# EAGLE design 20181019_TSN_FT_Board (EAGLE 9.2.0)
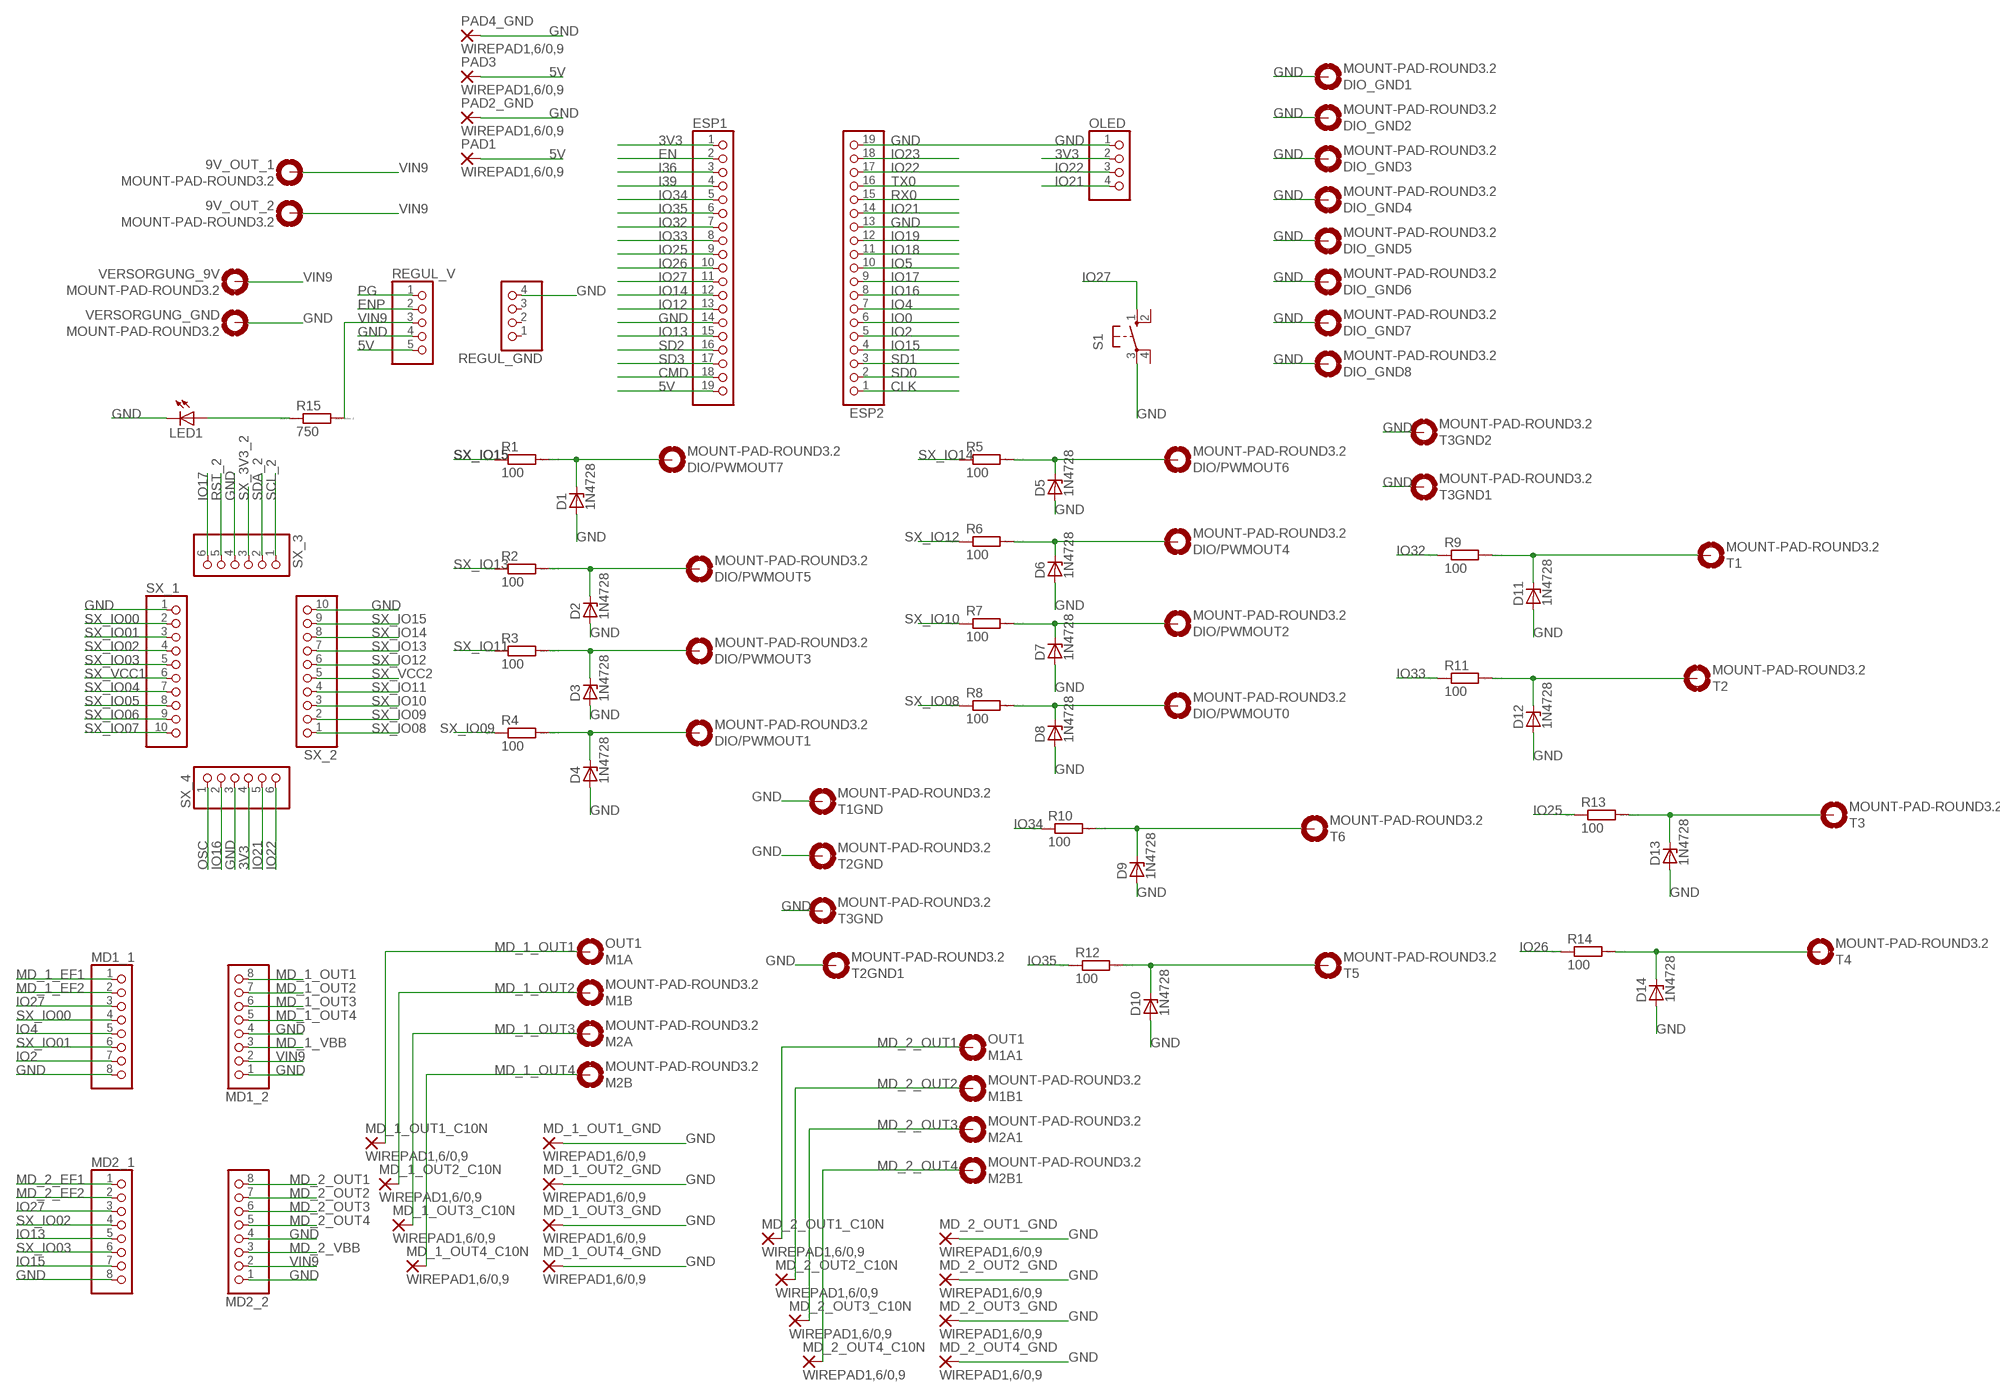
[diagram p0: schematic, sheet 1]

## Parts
9V_OUT_1  MOUNT-PAD-ROUND3.2  [3,2-PAD]
9V_OUT_2  MOUNT-PAD-ROUND3.2  [3,2-PAD]
D1  1N4728  [DO41Z10]
D2  1N4728  [DO41Z10]
D3  1N4728  [DO41Z10]
D4  1N4728  [DO41Z10]
D5  1N4728  [DO41Z10]
D6  1N4728  [DO41Z10]
D7  1N4728  [DO41Z10]
D8  1N4728  [DO41Z10]
D9  1N4728  [DO41Z10]
D10  1N4728  [DO41Z10]
D11  1N4728  [DO41Z10]
D12  1N4728  [DO41Z10]
D13  1N4728  [DO41Z10]
D14  1N4728  [DO41Z10]
DIO/PWMOUT0  MOUNT-PAD-ROUND3.2  [3,2-PAD]
DIO/PWMOUT1  MOUNT-PAD-ROUND3.2  [3,2-PAD]
DIO/PWMOUT2  MOUNT-PAD-ROUND3.2  [3,2-PAD]
DIO/PWMOUT3  MOUNT-PAD-ROUND3.2  [3,2-PAD]
DIO/PWMOUT4  MOUNT-PAD-ROUND3.2  [3,2-PAD]
DIO/PWMOUT5  MOUNT-PAD-ROUND3.2  [3,2-PAD]
DIO/PWMOUT6  MOUNT-PAD-ROUND3.2  [3,2-PAD]
DIO/PWMOUT7  MOUNT-PAD-ROUND3.2  [3,2-PAD]
DIO_GND1  MOUNT-PAD-ROUND3.2  [3,2-PAD]
DIO_GND2  MOUNT-PAD-ROUND3.2  [3,2-PAD]
DIO_GND3  MOUNT-PAD-ROUND3.2  [3,2-PAD]
DIO_GND4  MOUNT-PAD-ROUND3.2  [3,2-PAD]
DIO_GND5  MOUNT-PAD-ROUND3.2  [3,2-PAD]
DIO_GND6  MOUNT-PAD-ROUND3.2  [3,2-PAD]
DIO_GND7  MOUNT-PAD-ROUND3.2  [3,2-PAD]
DIO_GND8  MOUNT-PAD-ROUND3.2  [3,2-PAD]
ESP1  PINHD-1X19  [1X19]
ESP2  PINHD-1X19  [1X19]
LED1  LED3MM  [LED3MM]
M1A  OUT1  MOUNT-PAD-ROUND3.2  [3,2-PAD]
M1A1  OUT1  MOUNT-PAD-ROUND3.2  [3,2-PAD]
M1B  MOUNT-PAD-ROUND3.2  [3,2-PAD]
M1B1  MOUNT-PAD-ROUND3.2  [3,2-PAD]
M2A  MOUNT-PAD-ROUND3.2  [3,2-PAD]
M2A1  MOUNT-PAD-ROUND3.2  [3,2-PAD]
M2B  MOUNT-PAD-ROUND3.2  [3,2-PAD]
M2B1  MOUNT-PAD-ROUND3.2  [3,2-PAD]
MD1_1  PINHD-1X8  [1X08]
MD1_2  PINHD-1X8  [1X08]
MD2_1  PINHD-1X8  [1X08]
MD2_2  PINHD-1X8  [1X08]
MD_1_OUT1_C10N  WIREPAD1,6/0,9  [1,6/0,9]
MD_1_OUT1_GND  WIREPAD1,6/0,9  [1,6/0,9]
MD_1_OUT2_C10N  WIREPAD1,6/0,9  [1,6/0,9]
MD_1_OUT2_GND  WIREPAD1,6/0,9  [1,6/0,9]
MD_1_OUT3_C10N  WIREPAD1,6/0,9  [1,6/0,9]
MD_1_OUT3_GND  WIREPAD1,6/0,9  [1,6/0,9]
MD_1_OUT4_C10N  WIREPAD1,6/0,9  [1,6/0,9]
MD_1_OUT4_GND  WIREPAD1,6/0,9  [1,6/0,9]
MD_2_OUT1_C10N  WIREPAD1,6/0,9  [1,6/0,9]
MD_2_OUT1_GND  WIREPAD1,6/0,9  [1,6/0,9]
MD_2_OUT2_C10N  WIREPAD1,6/0,9  [1,6/0,9]
MD_2_OUT2_GND  WIREPAD1,6/0,9  [1,6/0,9]
MD_2_OUT3_C10N  WIREPAD1,6/0,9  [1,6/0,9]
MD_2_OUT3_GND  WIREPAD1,6/0,9  [1,6/0,9]
MD_2_OUT4_C10N  WIREPAD1,6/0,9  [1,6/0,9]
MD_2_OUT4_GND  WIREPAD1,6/0,9  [1,6/0,9]
OLED  PINHD-1X4  [1X04]
PAD1  WIREPAD1,6/0,9  [1,6/0,9]
PAD2_GND  WIREPAD1,6/0,9  [1,6/0,9]
PAD3  WIREPAD1,6/0,9  [1,6/0,9]
PAD4_GND  WIREPAD1,6/0,9  [1,6/0,9]
R1  100  R0207/10  [0207/10]
R2  100  R0207/10  [0207/10]
R3  100  R0207/10  [0207/10]
R4  100  R0207/10  [0207/10]
R5  100  R0207/10  [0207/10]
R6  100  R0207/10  [0207/10]
R7  100  R0207/10  [0207/10]
R8  100  R0207/10  [0207/10]
R9  100  R0207/10  [0207/10]
R10  100  R0207/10  [0207/10]
R11  100  R0207/10  [0207/10]
R12  100  R0207/10  [0207/10]
R13  100  R0207/10  [0207/10]
R14  100  R0207/10  [0207/10]
R15  750  R0207/10  [0207/10]
REGUL_GND  PINHD-1X4  [1X04]
REGUL_V  PINHD-1X5  [1X05]
S1  10-XX  [B3F-10XX]
SX_1  PINHD-1X10  [1X10]
SX_2  PINHD-1X10  [1X10]
SX_3  PINHD-1X6  [1X06]
SX_4  PINHD-1X6  [1X06]
T1  MOUNT-PAD-ROUND3.2  [3,2-PAD]
T1GND  MOUNT-PAD-ROUND3.2  [3,2-PAD]
T2  MOUNT-PAD-ROUND3.2  [3,2-PAD]
T2GND  MOUNT-PAD-ROUND3.2  [3,2-PAD]
T2GND1  MOUNT-PAD-ROUND3.2  [3,2-PAD]
T3  MOUNT-PAD-ROUND3.2  [3,2-PAD]
T3GND  MOUNT-PAD-ROUND3.2  [3,2-PAD]
T3GND1  MOUNT-PAD-ROUND3.2  [3,2-PAD]
T3GND2  MOUNT-PAD-ROUND3.2  [3,2-PAD]
T4  MOUNT-PAD-ROUND3.2  [3,2-PAD]
T5  MOUNT-PAD-ROUND3.2  [3,2-PAD]
T6  MOUNT-PAD-ROUND3.2  [3,2-PAD]
VERSORGUNG_9V  MOUNT-PAD-ROUND3.2  [3,2-PAD]
VERSORGUNG_GND  MOUNT-PAD-ROUND3.2  [3,2-PAD]

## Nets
3V3 [3V3]: ESP1.1 OLED.2 SX_4.4
5V [Bigger]: ESP1.19 PAD1.1(P) PAD3.1(P) REGUL_V.5
CLK: ESP2.1
CMD: ESP1.18
EN: ESP1.2
ENP: REGUL_V.2
GND [MOT_OUT]: D1.A D2.A D3.A D4.A D5.A D6.A D7.A D8.A D9.A D10.A D11.A D12.A D13.A D14.A DIO_GND1.BH3,2(MOUNT) DIO_GND2.BH3,2(MOUNT) DIO_GND3.BH3,2(MOUNT) DIO_GND4.BH3,2(MOUNT) DIO_GND5.BH3,2(MOUNT) DIO_GND6.BH3,2(MOUNT) DIO_GND7.BH3,2(MOUNT) DIO_GND8.BH3,2(MOUNT) ESP1.14 ESP2.13 ESP2.19 LED1.K(C) MD1_1.8 MD1_2.1 MD1_2.4 MD2_1.8 MD2_2.1 MD2_2.4 MD_1_OUT1_GND.1(P) MD_1_OUT2_GND.1(P) MD_1_OUT3_GND.1(P) MD_1_OUT4_GND.1(P) MD_2_OUT1_GND.1(P) MD_2_OUT2_GND.1(P) MD_2_OUT3_GND.1(P) MD_2_OUT4_GND.1(P) OLED.1 PAD2_GND.1(P) PAD4_GND.1(P) REGUL_GND.4 REGUL_V.4 S1.3(P) SX_1.1 SX_2.10 SX_3.4 SX_4.3 T1GND.BH3,2(MOUNT) T2GND1.BH3,2(MOUNT) T2GND.BH3,2(MOUNT) T3GND1.BH3,2(MOUNT) T3GND2.BH3,2(MOUNT) T3GND.BH3,2(MOUNT) VERSORGUNG_GND.BH3,2(MOUNT)
I36: ESP1.3
I39: ESP1.4
IO0: ESP2.6
IO2: ESP2.5 MD1_1.7
IO4: ESP2.7 MD1_1.5
IO5: ESP2.10
IO12: ESP1.13
IO13: ESP1.15 MD2_1.5
IO14: ESP1.12
IO15: ESP2.4 MD2_1.7
IO16: ESP2.8 SX_4.2
IO17: ESP2.9 SX_3.6
IO18: ESP2.11
IO19: ESP2.12
IO21: ESP2.14 OLED.4 SX_4.5
IO22: ESP2.17 OLED.3 SX_4.6
IO23: ESP2.18
IO25: ESP1.9 R13.1
IO26: ESP1.10 R14.1
IO27: ESP1.11 MD1_1.3 MD2_1.3 S1.1(S)
IO32: ESP1.7 R9.1
IO33: ESP1.8 R11.1
IO34: ESP1.5 R10.1
IO35: ESP1.6 R12.1
MD_1_EF1: MD1_1.1
MD_1_EF2: MD1_1.2
MD_1_OUT1 [Bigger]: M1A.BH3,2(MOUNT) MD1_2.8 MD_1_OUT1_C10N.1(P)
MD_1_OUT2 [Bigger]: M1B.BH3,2(MOUNT) MD1_2.7 MD_1_OUT2_C10N.1(P)
MD_1_OUT3 [Bigger]: M2A.BH3,2(MOUNT) MD1_2.6 MD_1_OUT3_C10N.1(P)
MD_1_OUT4 [Bigger]: M2B.BH3,2(MOUNT) MD1_2.5 MD_1_OUT4_C10N.1(P)
MD_1_VBB [MOT_OUT]: MD1_2.3
MD_2_EF1: MD2_1.1
MD_2_EF2: MD2_1.2
MD_2_OUT1 [Bigger]: M1A1.BH3,2(MOUNT) MD2_2.8 MD_2_OUT1_C10N.1(P)
MD_2_OUT2 [Bigger]: M1B1.BH3,2(MOUNT) MD2_2.7 MD_2_OUT2_C10N.1(P)
MD_2_OUT3 [Bigger]: M2A1.BH3,2(MOUNT) MD2_2.6 MD_2_OUT3_C10N.1(P)
MD_2_OUT4 [Bigger]: M2B1.BH3,2(MOUNT) MD2_2.5 MD_2_OUT4_C10N.1(P)
MD_2_VBB [MOT_OUT]: MD2_2.3
N$1: D5.C DIO/PWMOUT6.BH3,2(MOUNT) R5.2
N$2: D6.C DIO/PWMOUT4.BH3,2(MOUNT) R6.2
N$3: D7.C DIO/PWMOUT2.BH3,2(MOUNT) R7.2
N$4: D8.C DIO/PWMOUT0.BH3,2(MOUNT) R8.2
N$5: D1.C DIO/PWMOUT7.BH3,2(MOUNT) R1.2
N$6: D2.C DIO/PWMOUT5.BH3,2(MOUNT) R2.2
N$7: D3.C DIO/PWMOUT3.BH3,2(MOUNT) R3.2
N$8: D4.C DIO/PWMOUT1.BH3,2(MOUNT) R4.2
N$9: D9.C R10.2 T6.BH3,2(MOUNT)
N$10: LED1.A R15.1
N$12: D10.C R12.2 T5.BH3,2(MOUNT)
OSC: SX_4.1
PG: REGUL_V.1
RST_2: SX_3.5
RX0: ESP2.15
SCL_2: SX_3.1
SD0: ESP2.2
SD1: ESP2.3
SD2: ESP1.16
SD3: ESP1.17
SDA_2: SX_3.2
SX_3V3_2: SX_3.3
SX_IO00: MD1_1.4 SX_1.2
SX_IO01: MD1_1.6 SX_1.3
SX_IO02: MD2_1.4 SX_1.4
SX_IO03: MD2_1.6 SX_1.5
SX_IO04: SX_1.7
SX_IO05: SX_1.8
SX_IO06: SX_1.9
SX_IO07: SX_1.10
SX_IO08: R8.1 SX_2.1
SX_IO09: R4.1 SX_2.2
SX_IO10: R7.1 SX_2.3
SX_IO11: R3.1 SX_2.4
SX_IO12: R6.1 SX_2.6
SX_IO13: R2.1 SX_2.7
SX_IO14: R5.1 SX_2.8
SX_IO15: R1.1 SX_2.9
SX_IO17: D11.C R9.2 T1.BH3,2(MOUNT)
SX_IO18: D12.C R11.2 T2.BH3,2(MOUNT)
SX_IO19: D13.C R13.2 T3.BH3,2(MOUNT)
SX_IO20: D14.C R14.2 T4.BH3,2(MOUNT)
SX_VCC1: SX_1.6
SX_VCC2: SX_2.5
TX0: ESP2.16
VIN9 [MOT_OUT]: 9V_OUT_1.BH3,2(MOUNT) 9V_OUT_2.BH3,2(MOUNT) MD1_2.2 MD2_2.2 R15.2 REGUL_V.3 VERSORGUNG_9V.BH3,2(MOUNT)
Unconnected: REGUL_GND.1 REGUL_GND.2 REGUL_GND.3 S1.2(S1) S1.4(P1)

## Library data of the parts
9V_OUT_1 9V_OUT_2 DIO/PWMOUT0 DIO/PWMOUT1-DIO/PWMOUT7 DIO_GND1-DIO_GND8 M1A M1A1 M1B M1B1 M2A M2A1 M2B M2B1 T1 T1GND T2 T2GND T2GND1 T3 T3GND T3GND1 T3GND2 T4-T6 VERSORGUNG_9V VERSORGUNG_GND = Walter:MOUNT-PAD-ROUND: MOUNTING PAD, round
D1-D14 = diode:1N4728: Z DIODE
ESP1 = pinhead:PINHD-1X19: PIN HEADER
ESP2 = pinhead:PINHD-1X19: PIN HEADER; SPICEPREFIX: X
LED1 = led:LED: LED
MD1_1 MD1_2 MD2_1 MD2_2 = pinhead:PINHD-1X8: PIN HEADER
MD_1_OUT1_C10N MD_1_OUT1_GND MD_1_OUT2_C10N MD_1_OUT2_GND MD_1_OUT3_C10N MD_1_OUT3_GND MD_1_OUT4_C10N MD_1_OUT4_GND MD_2_OUT1_C10N MD_2_OUT1_GND MD_2_OUT2_C10N MD_2_OUT2_GND MD_2_OUT3_C10N MD_2_OUT3_GND MD_2_OUT4_C10N MD_2_OUT4_GND PAD1 PAD2_GND PAD3 PAD4_GND = wirepad:WIREPAD: Wire PAD connect wire on PCB
OLED REGUL_GND = pinhead:PINHD-1X4: PIN HEADER
R1-R15 = eagle-ltspice:R: RESISTOR, European symbol; SPICEMODEL: NONE; SPICEPREFIX: R
REGUL_V = pinhead:PINHD-1X5: PIN HEADER
S1 = switch-omron:10-XX: OMRON SWITCH; MPN: B3F-1000; OC_FARNELL: 176432; OC_NEWARK: 36M3542
SX_1 SX_2 = pinhead:PINHD-1X10: PIN HEADER
SX_3 SX_4 = pinhead:PINHD-1X6: PIN HEADER

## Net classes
1 MOT_OUT: width 0.6 mm
2 Bigger: width 0.6 mm
3 3V3: width 0.3 mm

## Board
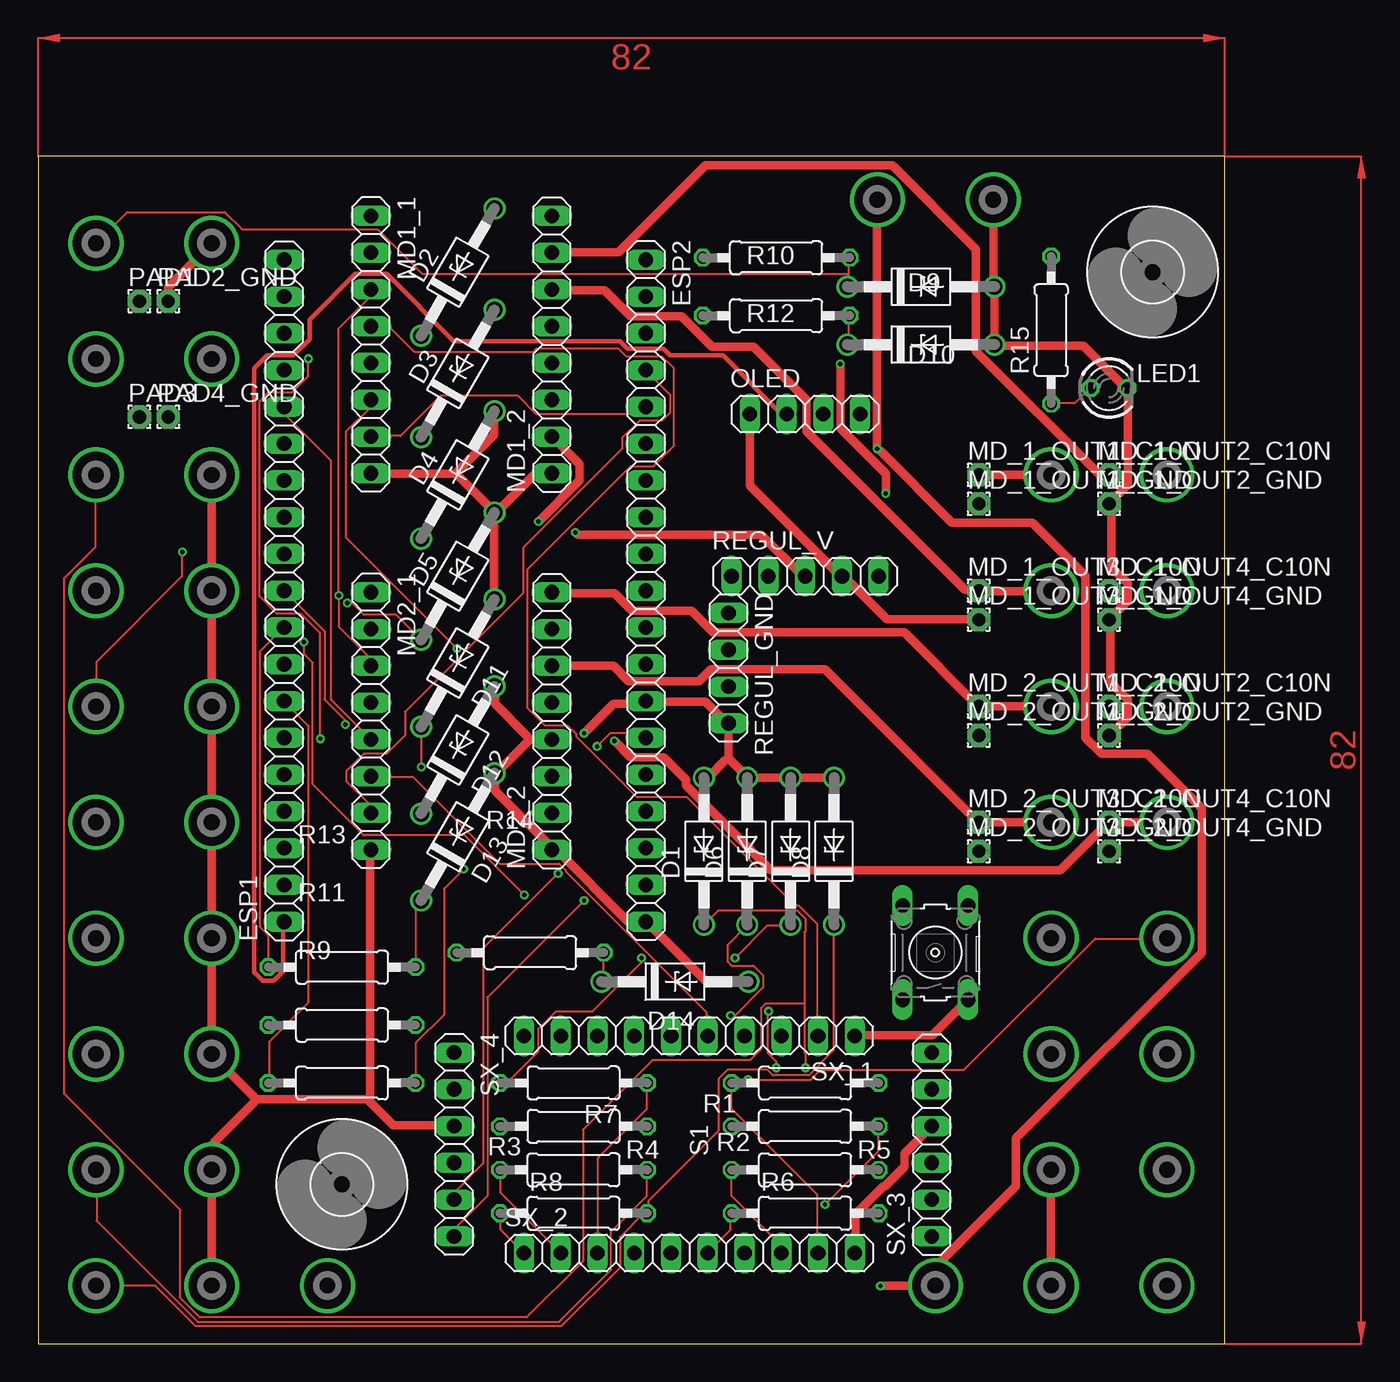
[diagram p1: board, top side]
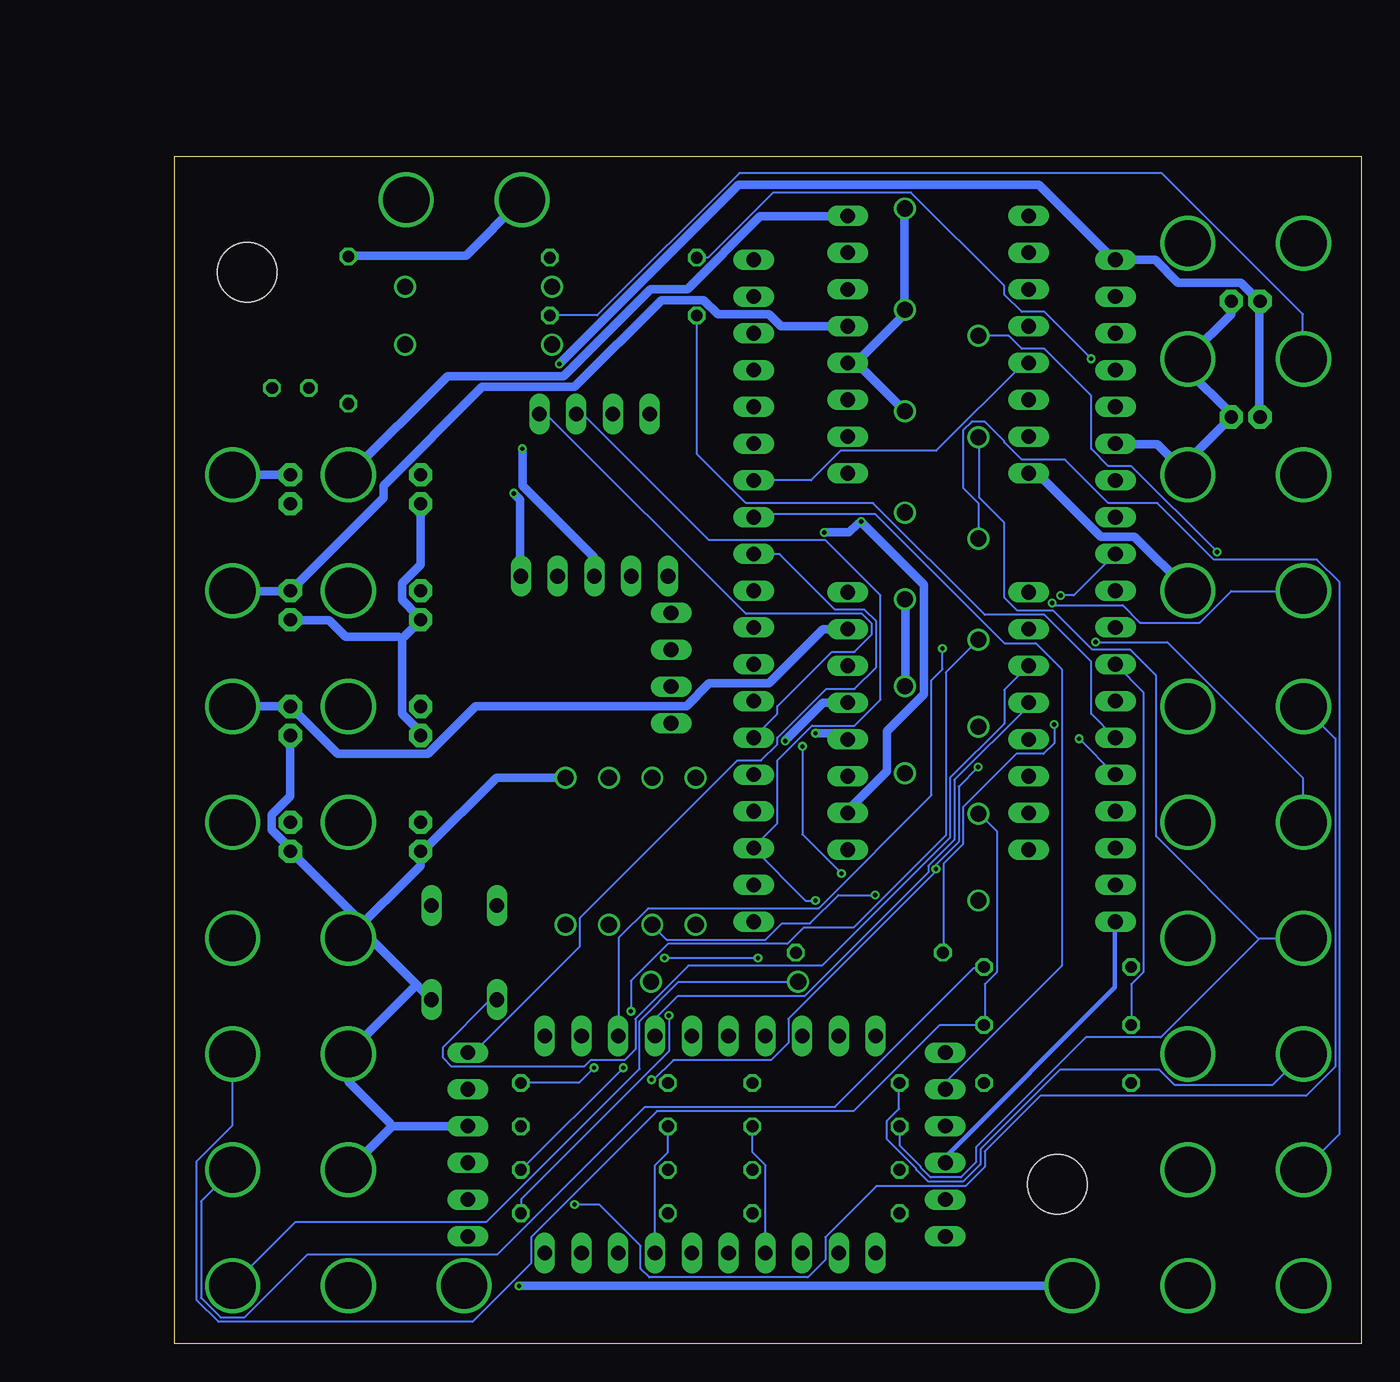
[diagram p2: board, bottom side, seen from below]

Size 82 x 82 mm. Coordinates in mm from the lower left corner, seen from the top.
Outline: 0,0 82,0 82,82 0,82 0,0
Copper layers (1+2+3*14+15+16): Top 0.035mm / dielectric 0.2mm / Route2 0.035mm / dielectric 0.36mm / Route3 0.035mm / dielectric 0.28mm / Route14 0.035mm / dielectric 0.36mm / Route15 0.035mm / dielectric 0.2mm / Bottom 0.035mm
Design rules "PCB-POOL Standard_ML6": minimum track width 0.15mm, minimum drill 0.3mm, track to track 0.15mm, track to pad 0.15mm, pad to pad 0.15mm, via to via 0.15mm, smd to smd 0.15mm, copper to edge 0.3mm, drill to drill 0.2mm, minimum pad ring 0.2mm, minimum via ring 0.15mm, stop-mask expansion 0.075mm, vias tented up to drill 0mil, thermal gap 0.2mm

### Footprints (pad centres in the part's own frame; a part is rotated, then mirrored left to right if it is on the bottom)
3,2-PAD = drill 3.2 pad 3.81: BH3,2 0,0
DO41Z10 = drill 1.118: A 5.08,0; C -5.08,0
1X19 = drill 1.016 long: 1 -22.86,0; 2 -20.32,0; 3 -17.78,0; 4 -15.24,0; 5 -12.7,0; 6 -10.16,0; 7 -7.62,0; 8 -5.08,0; 9 -2.54,0; 10 0,0; 11 2.54,0; 12 5.08,0; 13 7.62,0; 14 10.16,0; 15 12.7,0; 16 15.24,0; 17 17.78,0; 18 20.32,0; 19 22.86,0
LED3MM = drill 0.813 octagon: A -1.27,0; K 1.27,0
1X08 = drill 1.016 long: 1 -8.89,0; 2 -6.35,0; 3 -3.81,0; 4 -1.27,0; 5 1.27,0; 6 3.81,0; 7 6.35,0; 8 8.89,0
1,6/0,9 = drill 0.914 pad 1.6 octagon: 1 0,0
1X04 = drill 1.016 long: 1 -3.81,0; 2 -1.27,0; 3 1.27,0; 4 3.81,0
0207/10 = drill 0.813 octagon: 1 -5.08,0; 2 5.08,0
1X05 = drill 1.016 long: 1 -5.08,0; 2 -2.54,0; 3 0,0; 4 2.54,0; 5 5.08,0
B3F-10XX = drill 1.016 long: 1 -3.251,2.261; 2 3.251,2.261; 3 -3.251,-2.261; 4 3.251,-2.261
1X10 = drill 1.016 long: 1 -11.43,0; 2 -8.89,0; 3 -6.35,0; 4 -3.81,0; 5 -1.27,0; 6 1.27,0; 7 3.81,0; 8 6.35,0; 9 8.89,0; 10 11.43,0
1X06 = drill 1.016 long: 1 -6.35,0; 2 -3.81,0; 3 -1.27,0; 4 1.27,0; 5 3.81,0; 6 6.35,0
4,1 = hole 4.1: 0,0

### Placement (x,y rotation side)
9V_OUT_1  20,4 0 top
9V_OUT_2  62,4 0 top
D1  46,34 90 top
D2  29,74 60 top
D3  29,67 60 top
D4  29,60 60 top
D5  29,53 60 top
D6  49,34 90 top
D7  52,34 90 top
D8  55,34 90 top
D9  61,73 0 top
D10  61,69 0 top
D11  29,47 60 top
D12  29,41 60 top
D13  29,35 60 top
D14  44,25 0 top
DIO/PWMOUT0  4,4 0 top
DIO/PWMOUT1  4,12 0 top
DIO/PWMOUT2  4,20 0 top
DIO/PWMOUT3  4,28 0 top
DIO/PWMOUT4  4,36 0 top
DIO/PWMOUT5  4,44 0 top
DIO/PWMOUT6  4,52 0 top
DIO/PWMOUT7  4,60 0 top
DIO_GND1  12,52 0 top
DIO_GND2  12,60 180 top
DIO_GND3  12,44 90 top
DIO_GND4  12,36 0 top
DIO_GND5  12,28 0 top
DIO_GND6  12,20 0 top
DIO_GND7  12,12 0 top
DIO_GND8  12,4 180 top
ESP1  17,52 90 top
ESP2  42,52 270 top
LED1  74,66 0 top
M1A  70,60 0 top
M1A1  70,44 0 top
M1B  78,60 0 top
M1B1  78,44 0 top
M2A  70,52 0 top
M2A1  70,36 0 top
M2B  78,52 0 top
M2B1  78,36 0 top
MD1_1  23,69 270 top
MD1_2  35.5,69 90 top
MD2_1  23,43 270 top
MD2_2  35.5,43 90 top
MD_1_OUT1_C10N  65,60 0 top
MD_1_OUT1_GND  65,58 0 top
MD_1_OUT2_C10N  74,60 0 top
MD_1_OUT2_GND  74,58 0 top
MD_1_OUT3_C10N  65,52 0 top
MD_1_OUT3_GND  65,50 0 top
MD_1_OUT4_C10N  74,52 0 top
MD_1_OUT4_GND  74,50 0 top
MD_2_OUT1_C10N  65,44 0 top
MD_2_OUT1_GND  65,42 0 top
MD_2_OUT2_C10N  74,44 0 top
MD_2_OUT2_GND  74,42 0 top
MD_2_OUT3_C10N  65,36 0 top
MD_2_OUT3_GND  65,34 0 top
MD_2_OUT4_C10N  74,36 0 top
MD_2_OUT4_GND  74,34 0 top
OLED  52.99,64.2 0 top
PAD1  7,72 0 top
PAD2_GND  9,72 0 top
PAD3  7,64 0 top
PAD4_GND  9,64 0 top
R1  53,18 0 top
R2  53,15 0 top
R3  37,15 180 top
R4  37,12 0 top
R5  53,12 0 top
R6  53,9 0 top
R7  37,18 180 top
R8  37,9 0 top
R9  21,18 0 top
R10  51,75 0 top
R11  21,22 0 top
R12  51,71 0 top
R13  21,26 0 top
R14  34,27 0 top
R15  70,70 90 top
REGUL_GND  47.7,46.65 270 top
REGUL_V  53,53 0 top
S1  62,27 90 top
SX_1  45,21.25 180 top
SX_2  45,6.25 0 top
SX_3  61.75,13.75 90 top
SX_4  28.75,13.75 270 top
T1  78,28 0 top
T1GND  70,20 90 top
T2  78,20 0 top
T2GND  70,28 0 top
T2GND1  70,4 0 top
T3  78,12 0 top
T3GND  70,12 0 top
T3GND1  12,68 0 top
T3GND2  12,76 90 top
T4  78,4 0 top
T5  4,68 0 top
T6  4,76 0 top
U$1  [4,1]  77,74 0 top
U$2  [4,1]  21,11 0 top
VERSORGUNG_9V  58,79 0 top
VERSORGUNG_GND  66,79 0 top

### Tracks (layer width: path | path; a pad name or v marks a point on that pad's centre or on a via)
3V3
  Top 0.3: OLED.2 51.38,64.2 47.33,68.25 43.65,68.25 43.2,68.7 40.73,68.7 40.2,69.22 28.73,69.22 24.07,73.88 21.9,73.88 18.75,70.72 18.75,69.38 17.62,68.25 15.82,68.25 14.93,67.35 14.93,25.65 15.53,25.05 16.27,25.05 16.95,25.73 16.95,29.1 ESP1.1
  Bottom 0.3: SX_4.4 28.73,12.53 28.73,12.9 17.02,24.6 17.02,29.1 ESP1.1
5V  (via drill 0.3)
  Top 0.6: v58.58,58.73 58.58,60.08 55.42,63.23 v55.42,67.65
  Bottom 0.6: v58.58,58.73 58.12,58.27 58.12,53.02 REGUL_V.5 | v55.42,67.65 43.05,80.03 22.27,80.03 17.25,75 ESP1.19 16.95,74.85 14.25,74.85 12.68,73.28 8.32,73.28 7.05,72 PAD1.1 7.05,71.78 7.05,64.05 PAD3.1
GND  (via drill 0.3)
  Top 0.6: VERSORGUNG_GND.BH3,2 66,73.28 D9.A 66.08,72.97 D10.A 66.38,68.92 72.22,68.92 75,66.15 LED1.K 75.3,66 75.3,59.33 74.03,58.05 MD_1_OUT2_GND.1 74.17,57.75 74.17,53.62 75.3,52.5 75.3,51.3 MD_1_OUT4_GND.1 74.1,49.73 74.1,45.67 75.3,44.48 75.3,43.27 74.03,42 MD_2_OUT2_GND.1 | MD_1_OUT3_GND.1 64.95,50.02 58.65,50.02 55.73,52.95 55.58,52.95 REGUL_V.4 55.27,53.17 49.2,59.25 49.2,64.2 OLED.1 | SX_2.10 56.48,6.3 56.48,8.93 58.42,10.88 58.5,10.88 59.85,12.22 59.85,13.12 61.73,15 SX_3.4 | T2GND1.BH3,2 69.97,4.05 69.97,12 T3GND.BH3,2 | 47.7,40.42 REGUL_GND.4 47.48,42.98 46.12,44.33 42,44.33 ESP2.13 41.77,44.17 39.75,44.17 v37.73,42.15 | 47.7,40.42 48.98,39.15 D6.A 49.27,39.08 51.98,39.08 D7.A 52.27,39.08 54.98,39.08 D8.A | D1.A 46.05,39.15 46.35,39.15 47.48,40.27 47.7,40.42 | SX_1.1 56.48,21.3 61.8,21.3 64.2,23.7 S1.3 | 33.98,41.7 35.48,41.7 MD2_2.4 | 33.98,41.7 31.8,39.52 D13.A 31.57,39.38 31.57,38.17 35.48,34.27 35.48,34.12 MD2_2.1 35.77,34.12 40.73,29.18 42,29.18 ESP2.19 42.23,28.95 46.12,25.05 49.05,25.05 D14.A | D12.A 31.57,45.38 31.57,44.17 33.83,41.92 33.98,41.7 | 28.88,60.08 23.02,60.08 MD1_1.8 | 28.88,60.08 31.5,57.45 D5.A | MD1_2.1 35.48,60.08 34.35,60.08 31.8,57.52 D5.A | D11.A 31.5,51.45 31.5,57.15 D5.A | D4.A 31.5,64.35 31.5,62.77 29.02,60.3 28.88,60.08 | PAD2_GND.1 9,72.97 12,75.97 T3GND2.BH3,2 | DIO_GND8.BH3,2 DIO_GND7.BH3,2 12.15,12.22 12.15,13.88 14.93,16.65 15.07,16.88 | 22.76,16.84 22.73,16.88 15.07,16.88 | 22.76,16.84 24.52,15.07 28.73,15.07 SX_4.3 | 15.07,16.88 12,19.95 DIO_GND6.BH3,2 DIO_GND5.BH3,2 DIO_GND4.BH3,2 DIO_GND3.BH3,2 DIO_GND1.BH3,2 DIO_GND2.BH3,2
  Top 0.6: MD2_1.8 22.95,34.05 22.95,17.02 22.76,16.84
  Bottom 0.6: 66.3,48.67 66.3,43.5 65.03,42.23 65.03,42 MD_2_OUT1_GND.1 | 66.3,48.67 65.03,49.95 MD_1_OUT3_GND.1 65.17,50.25 66.3,51.38 66.3,52.5 65.03,53.77 65.03,57.98 MD_1_OUT1_GND.1 | MD_1_OUT4_GND.1 73.95,49.95 71.33,49.95 70.2,48.83 66.53,48.83 66.3,48.67 | 66.97,15 61.8,15 SX_3.4 | 66.97,15 69.97,12 T3GND.BH3,2 | 66.97,15 67.12,15.22 69.97,18.07 69.97,19.95 T1GND.BH3,2 69.83,20.25 65.29,24.79 | T2GND.BH3,2 69.97,28.05 65.03,33 65.03,33.98 MD_2_OUT3_GND.1 64.72,34.12 59.77,39.08 55.05,39.08 D8.A | T2GND.BH3,2 69.15,29.18 73.95,33.98 MD_2_OUT4_GND.1 74.1,34.27 75.3,35.48 75.3,36.52 74.03,37.8 74.03,42 MD_2_OUT2_GND.1 | 65.29,24.79 69.08,28.57 T2GND.BH3,2 | 65.29,24.79 64.28,23.77 S1.3 | D4.A 31.57,64.42 34.88,67.72 35.48,67.72 MD1_2.4 34.73,67.95 31.57,71.1 31.57,71.33 D3.A 31.57,71.7 31.57,78.38 D2.A | D12.A 31.5,45.45 31.5,51.38 D11.A | ESP1.14 16.95,62.1 14.1,62.1 DIO_GND2.BH3,2 12.3,60.67 9,63.98 PAD4_GND.1 9.07,64.28 12,67.2 T3GND1.BH3,2 11.85,68.25 9,71.1 PAD2_GND.1 | MD1_1.8 22.95,60.08 22.35,60.08 18,55.73 15.68,55.73 12,52.05 DIO_GND1.BH3,2 | v37.73,42.15 35.92,42.15 35.55,41.77 MD2_2.4
IO2
  Top 0.15: MD1_1.7 23.02,62.7 25.05,62.7 27.82,65.47 33.15,65.47 34.42,64.2 41.55,64.2 42,64.65 ESP2.5
IO4
  Bottom 0.15: ESP2.7 38.02,59.62 36,61.65 29.4,61.65 23.32,67.72 23.02,67.72 MD1_1.5
IO13
  Top 0.15: ESP1.15 17.02,64.65 17.02,64.2 20.25,60.98 20.25,44.48 22.95,41.77 MD2_1.5
IO15
  Top 0.15: MD2_1.7 22.95,36.67 22.95,37.2 21.3,38.85 21.3,39.52 22.5,40.73 24.07,40.73 25.35,42 25.35,43.65 33.52,51.83 33.52,54.98 40.35,61.8 40.35,62.55 41.55,63.75 43.12,63.75 43.65,64.28 43.65,65.55 42,67.2 ESP2.4
IO16
  Bottom 0.15: SX_4.2 28.73,17.62 28.73,18.07 20.7,26.1 20.7,46.58 22.5,48.38 24.68,48.38 33.6,57.3 41.85,57.3 42,57.15 ESP2.8
IO17
  Bottom 0.15: SX_3.6 61.35,20.1 54,27.45 54,29.4 43.12,40.27 41.48,40.27 40.35,41.4 40.35,41.85 36.98,45.23 35.02,45.23 33.52,46.73 33.52,49.88 34.35,50.7 36.38,50.7 40.2,54.52 42,54.52 ESP2.9
IO21  (via drill 0.3)
  Top 0.15: v35.92,32.48 30.75,27.3 30.75,12.45 28.8,10.5 28.8,9.97 SX_4.5 | v38.62,41.25 39.52,42.15 41.7,42.15 ESP2.14
  Bottom 0.15: v35.92,32.48 38.62,35.17 v38.62,41.25 | OLED.4 56.33,64.2 42.52,50.4 34.5,50.4 33.83,49.73 33.83,48.98 35.02,47.77 36.6,47.77 40.35,44.02 40.35,43.5 ESP2.14
IO22  (via drill 0.3)
  Top 0.15: v37.73,30.6 31.05,23.93 31.05,10.2 28.8,7.95 28.8,7.42 SX_4.6
  Bottom 0.15: v37.73,30.6 38.4,30.6 42,34.2 ESP2.17 42,34.27 40.35,35.92 40.35,40.27 37.95,42.67 35.02,42.67 33.23,44.48 33.23,51.67 37.05,55.5 45.08,55.5 53.77,64.2 OLED.3
IO25
  Top 0.15: R13.1 15.9,26.02 15.9,28.2 15.3,28.8 15.3,47.77 16.95,49.42 ESP1.9
IO26  (via drill 0.3)
  Top 0.15: v21.23,42.75 21.23,43.05 19.8,44.48 19.8,49.2 ESP1.10
  Bottom 0.15: v21.23,42.75 21.23,41.48 21.98,40.73 23.85,40.73 27.52,37.05 27.52,34.5 28.88,33.15 28.88,27 R14.1
IO27  (via drill 0.3)
  Top 0.15: MD2_1.3 22.95,46.88 22.95,47.33 20.77,49.5 v20.77,51.67 20.77,70.12 22.95,72.3 22.95,72.75 MD1_1.3
  Bottom 0.15: v20.77,51.67 19.88,51.67 17.02,54.52 ESP1.11 | S1.1 59.77,23.7 60.23,23.7 63.45,20.48 63.45,19.73 62.85,19.12 53.7,19.12 53.25,19.57 50.92,19.57 50.17,20.32 50.17,22.43 46.5,26.1 37.27,26.1 28.43,34.95 28.43,39.08 24.68,42.83 24.68,45.15 23.02,46.8 MD2_1.3
IO32
  Top 0.15: R9.1 15.97,18 15.97,20.85 18.68,23.55 18.68,42.67 17.02,44.33 ESP1.7
IO33
  Bottom 0.15: R11.1 15.9,22.05 15.9,24.82 15.07,25.65 15.07,45 16.95,46.88 ESP1.8
IO34  (via drill 0.3)
  Top 0.15: v18.68,68.03 18.68,66.83 17.55,65.7 15.9,65.7 15.3,65.1 15.3,51.6 16.5,50.4 18.15,50.4 19.5,49.05 v19.5,41.77
  Bottom 0.15: R10.1 45.15,75 40.65,79.5 31.12,79.5 24.68,73.05 24.68,72.45 23.48,71.25 21.9,71.25 v18.68,68.03 | v19.5,41.77 17.02,39.3 ESP1.5
IO35
  Bottom 0.15: R12.1 45.9,70.95 45.9,61.42 42.52,58.05 33.75,58.05 26.02,50.33 21.9,50.33 18.68,47.1 18.68,43.5 17.02,41.85 ESP1.6
MD_1_OUT1
  Top 0.6: M1A.BH3,2 MD_1_OUT1_C10N.1
  Bottom 0.6: MD1_2.8 35.55,77.85 41.55,77.85 46.58,72.83 49.12,72.83 55.12,66.83 63.15,66.83 69.97,60 M1A.BH3,2
MD_1_OUT2
  Top 0.6: MD_1_OUT2_C10N.1 73.35,60 64.8,68.55 64.8,75.6 59.02,81.38 46.12,81.38 40.12,75.38 35.55,75.38 MD1_2.7
  Bottom 0.6: MD_1_OUT2_C10N.1 M1B.BH3,2
MD_1_OUT3
  Top 0.6: MD1_2.6 35.55,72.75 39.15,72.75 40.95,70.95 44.48,70.95 46.58,68.85 49.42,68.85 53.1,65.17 53.1,63 64.05,52.05 64.95,52.05 MD_1_OUT3_C10N.1 65.25,51.98 69.97,51.98 M2A.BH3,2
MD_1_OUT4
  Bottom 0.6: MD1_2.5 35.55,70.28 40.12,70.28 40.95,71.1 44.48,71.1 45.45,72.08 48.38,72.08 54.38,66.08 60.75,66.08 67.58,59.25 67.58,58.42 MD_1_OUT4_C10N.1 74.25,51.98 78,51.98 M2B.BH3,2
MD_2_OUT1
  Top 0.6: MD2_2.8 35.55,51.83 39.83,51.83 41.02,50.62 45.15,50.62 46.65,49.12 59.85,49.12 64.95,44.02 MD_2_OUT1_C10N.1 65.25,44.02 69.97,44.02 M1A1.BH3,2
MD_2_OUT2
  Bottom 0.6: MD2_2.7 37.2,49.35 40.95,45.6 45.08,45.6 46.65,44.02 61.2,44.02 64.5,40.73 70.72,40.73 MD_2_OUT2_C10N.1 74.25,44.02 78,44.02 M1B1.BH3,2
MD_2_OUT3
  Top 0.6: MD2_2.6 35.55,46.8 39.75,46.8 40.8,45.75 45.67,45.75 46.5,46.58 54.38,46.58 64.95,36 MD_2_OUT3_C10N.1 M2A1.BH3,2
MD_2_OUT4  (via drill 0.3)
  Top 0.6: v39.83,41.62 40.95,40.5 43.2,40.5 44.77,38.92 44.77,38.55 50.62,32.7 70.65,32.7 73.95,36 MD_2_OUT4_C10N.1 M2B1.BH3,2
  Bottom 0.6: v39.83,41.62 37.2,44.25 35.55,44.25 MD2_2.5
N$1  (via drill 0.3)
  Top 0.15: v51,19.05 51,19.5 50.4,20.1 50.4,22.88 v50.48,22.95 | v21.38,51.15 21.68,51.15 22.5,50.33 24.75,50.33 26.4,48.67 D5.C
  Bottom 0.15: v51,19.05 58.05,12 R5.2 | v50.48,22.95 50.48,25.05 47.92,27.6 39.67,27.6 38.55,28.73 35.1,28.73 28.73,35.1 28.73,46.35 26.48,48.6 D5.C | v21.38,51.15 21.23,51 16.5,51 15.3,49.8 11.18,49.8 9,51.98 4.05,51.98 DIO/PWMOUT6.BH3,2
N$2  (via drill 0.3)
  Top 0.15: v47.85,22.65 48.15,22.65 50.1,24.6 50.1,25.43 49.42,26.1 47.92,26.1 47.62,26.4 47.62,27.52 48.98,28.88 D6.C | v18.38,48.45 18.38,47.62 18.98,47.02 18.98,38.62 22.5,35.1 29.48,35.1 v33.6,30.98
  Bottom 0.15: v47.85,22.65 47.85,20.18 58.05,9.97 58.05,9 R6.2 | v18.38,48.45 13.43,48.45 4.05,39.08 4.05,36 DIO/PWMOUT4.BH3,2 | v33.6,30.98 36.15,30.98 38.1,29.02 40.05,29.02 41.17,27.9 48,27.9 48.98,28.88 D6.C
N$3  (via drill 0.3)
  Top 0.15: v48.15,26.62 50.4,28.88 51.98,28.88 D7.C | v41.7,26.62 41.7,26.32 38.33,22.95 35.77,22.95 34.58,21.75 34.58,20.18 32.4,18 R7.2
  Bottom 0.15: DIO/PWMOUT2.BH3,2 6.15,17.85 12.9,17.85 13.95,18.9 20.85,18.9 26.32,13.43 26.32,12.38 27.52,11.18 29.93,11.18 30.75,12 30.75,12.07 32.77,14.1 32.77,15.38 31.95,16.2 31.95,18 R7.2 | v41.7,26.62 v48.15,26.62
N$4
  Top 0.15: D8.C 54.98,28.88 54.98,20.25 53.25,18.52 50.77,18.52 50.4,18.9 47.62,18.9 47.02,18.3 47.02,14.7 42.15,9.82 42.15,9 R8.2 41.85,9 40.2,7.35 40.2,5.25 36.15,1.2 10.88,1.2 8.1,3.98 4.05,3.98 DIO/PWMOUT0.BH3,2
N$5  (via drill 0.3)
  Top 0.15: v53.02,19.05 53.02,20.02 52.95,20.1 52.95,23.48 | 52.95,23.48 52.95,28.43 53.02,28.5 53.02,29.32 52.42,29.93 47.02,29.93 46.05,28.95 D1.C | 52.95,23.48 50.25,23.48 49.95,23.18 49.95,20.32 49.2,19.57 42.45,19.57 37.65,14.78 37.65,5.7 33.75,1.8 11.18,1.8 9.82,3.15 9.82,9.22 1.8,17.25 1.8,52.88 3.98,55.05 3.98,60 DIO/PWMOUT7.BH3,2
  Bottom 0.15: R1.2 54.08,18 v53.02,19.05
N$6  (via drill 0.3)
  Top 0.15: v54.38,9.6 58.05,13.28 58.05,15 R2.2 | v9.97,54.67 9.97,53.02 4.05,47.1 4.05,44.02 DIO/PWMOUT5.BH3,2
  Bottom 0.15: v54.38,9.6 52.65,9.6 49.8,6.75 49.8,5.17 49.2,4.58 38.25,4.58 37.05,5.78 37.05,7.35 33.52,10.88 27.38,10.88 26.02,12.22 26.02,13.28 22.2,17.1 3.83,17.1 1.8,19.12 1.8,41.77 3.98,43.95 DIO/PWMOUT5.BH3,2 | v9.97,54.67 15.9,60.6 17.48,60.6 18.68,61.8 18.68,65.47 21.9,68.7 23.48,68.7 24.38,69.6 26.4,69.6 D2.C
N$7
  Bottom 0.15: 7.09,27.94 7.05,27.98 4.05,27.98 DIO/PWMOUT3.BH3,2 | 7.09,27.94 13.88,21.15 19.05,21.15 26.62,13.57 26.62,12.53 27.68,11.47 29.77,11.47 30.45,12.15 30.45,12.22 31.88,13.65 31.88,15 R3.2 | 7.09,27.94 14.18,35.02 14.18,46.12 15.97,47.92 18.6,47.92 21.3,50.62 23.77,50.62 24.68,51.52 24.68,56.7 26.4,58.42 26.4,62.55 D3.C
N$8
  Top 0.15: R4.2 42.08,10.2 39.6,7.72 39.6,5.1 36,1.5 11.03,1.5 4.05,8.47 4.05,12 DIO/PWMOUT1.BH3,2
  Bottom 0.15: D4.C 26.48,55.65 26.48,58.05 27.52,59.1 27.52,63.08 26.93,63.67 26.02,63.67 24.68,62.33 24.68,62.25 23.48,61.05 20.48,61.05 17.48,58.05 14.1,58.05 10.2,54.15 3.08,54.15 1.5,52.58 1.5,14.47 3.98,12 DIO/PWMOUT1.BH3,2
N$9
  Top 0.15: 56.02,73.88 56.02,73.12 55.95,73.05 D9.C | 56.02,73.88 56.02,75 R10.2 | 56.02,73.88 26.55,73.88 23.48,76.95 14.1,76.95 12.9,78.15 6.15,78.15 T6.BH3,2
N$10
  Top 0.15: R15.1 70.05,64.95 71.62,64.95 72.67,66 LED1.A
N$12
  Top 0.15: R12.2 56.02,70.95 56.02,69.08 55.95,69 D10.C
  Bottom 0.15: R12.2 56.02,71.03 52.8,71.03 42.98,80.85 13.8,80.85 4.05,71.1 4.05,68.03 T5.BH3,2
SX_IO00
  Top 0.15: MD1_1.4 23.02,70.2 24.3,70.2 26.02,68.47 34.2,68.47 34.42,68.7 40.12,68.7 40.65,68.17 43.12,68.17 43.95,67.35 43.95,62.02 42.52,60.6 40.95,60.6 33.83,53.48 33.83,43.88 35.02,42.67 36.6,42.67 37.2,42.08 37.2,41.92 41.4,37.73 44.85,37.73 52.35,30.23 52.58,30.23 53.85,28.95 53.85,21.3 SX_1.2
SX_IO01  (via drill 0.3)
  Top 0.15: v28.95,48 21.3,55.65 21.3,63 22.95,64.65 22.95,65.17 MD1_1.6
  Bottom 0.15: v28.95,48 28.95,46.58 29.7,45.83 29.7,37.88 37.5,30.07 49.27,30.07 51.3,28.05 51.3,21.3 SX_1.3
SX_IO02
  Bottom 0.15: SX_1.4 48.75,21.3 48.75,22.5 47.25,24 38.48,24 29.93,32.55 29.93,33 28.12,34.8 28.12,38.92 23.02,44.02 23.02,44.25 MD2_1.4
SX_IO03
  Top 0.15: SX_1.5 46.2,21.3 46.2,22.88 36.45,32.62 36.45,32.7 36,33.15 31.88,33.15 25.88,39.15 23.02,39.15 MD2_1.6
SX_IO08
  Top 0.15: R8.1 31.95,9 31.95,7.88 33.52,6.3 SX_2.1
SX_IO09
  Top 0.15: R4.1 31.95,12 31.95,10.43 36.08,6.3 SX_2.2
SX_IO10
  Top 0.15: R7.1 42.08,16.2 38.7,12.82 38.7,6.3 SX_2.3
SX_IO11
  Bottom 0.15: R3.1 42.08,13.2 41.17,12.3 41.17,6.3 SX_2.4
SX_IO12
  Top 0.15: R6.1 47.85,9 47.85,7.88 46.27,6.3 SX_2.6
SX_IO13
  Bottom 0.15: R2.1 47.92,13.2 48.83,12.3 48.83,6.3 SX_2.7
SX_IO14
  Top 0.15: R5.1 47.92,10.2 51.3,6.83 51.3,6.3 SX_2.8
SX_IO15
  Top 0.15: R1.1 47.92,16.2 53.85,10.28 53.85,6.3 SX_2.9
SX_IO17  (via drill 0.3)
  Top 0.15: v29.4,32.77 28.05,31.43 28.05,22.73 26.1,20.77 26.1,18 R9.2 | v26.48,39.83 26.48,42.6 D11.C | v49.05,18.23 53.4,18.23 54.08,18.9 63.98,18.9 73.05,27.98 78,27.98 T1.BH3,2
  Bottom 0.15: v26.48,39.83 27.82,38.48 27.82,34.65 29.4,33.08 v29.4,32.77 29.4,32.62 39.6,22.43 39.6,20.77 40.8,19.57 47.55,19.57 48.9,18.23 v49.05,18.23
SX_IO18
  Bottom 0.15: D12.C 26.4,36.6 25.2,35.4 25.2,25.65 26.02,24.82 26.02,22.05 R11.2 26.1,21.98 29.18,21.98 35.1,16.05 48.67,16.05 57.38,7.35 57.38,5.55 61.42,1.5 78.97,1.5 80.47,3 80.47,12.6 78,15.07 T2.BH3,2
SX_IO19
  Top 0.15: R13.2 26.1,26.02 26.1,30.3 26.4,30.6 D13.C
  Bottom 0.15: T3.BH3,2 80.17,9.82 80.17,3.15 78.83,1.8 77.17,1.8 72.83,6.15 59.7,6.15 49.5,16.35 36.38,16.35 26.77,25.95 26.1,25.95 R13.2
SX_IO20
  Top 0.15: R14.2 39.08,25.2 38.92,25.05 D14.C
  Bottom 0.15: D14.C 38.92,24.98 47.17,24.98 49.88,22.27 49.88,18.98 60.45,8.4 73.65,8.4 78,4.05 T4.BH3,2
VIN9  (via drill 0.3)
  Top 0.6: v58.2,3.98 61.95,3.98 9V_OUT_2.BH3,2 62.1,4.28 62.1,5.4 67.58,10.88 67.58,14.18 80.4,27 80.4,36.98 76.65,40.73 73.5,40.73 72.38,41.85 72.38,53.02 68.7,56.7 63.15,56.7 58.2,61.65 v57.98,61.8 57.98,78.97 VERSORGUNG_9V.BH3,2 | v34.58,56.77 37.42,59.62 37.42,60.75 35.55,62.62 MD1_2.2 | v37.12,56.02 37.27,55.88 49.95,55.88 52.8,53.02 52.95,53.02 REGUL_V.3
  Bottom 0.6: v58.2,3.98 20.02,3.98 9V_OUT_1.BH3,2 | R15.2 69.97,75.15 61.88,75.15 58.05,78.97 VERSORGUNG_9V.BH3,2 | MD2_2.2 35.48,36.67 35.48,36.83 32.77,39.52 32.77,42.3 30.23,44.85 30.23,52.42 v34.58,56.77 34.8,56.62 35.4,56.02 v37.12,56.02 | v57.98,61.8 57.98,59.25 53.02,54.3 53.02,53.02 REGUL_V.3
(copper drawn outside any net)
  shapes: Top area x2

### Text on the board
Beschriftung: GPI | GND | 9V | GND | max. 3,3V! | DIO | max. 5V! | Motoren 0 - 3 | GND | Encoder | max. 3,3V! | 9V out | 9V out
